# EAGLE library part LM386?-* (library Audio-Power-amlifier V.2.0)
Low Voltage Audio Power Amplifier Source: http://cache.national.com/ds/LM/LM386.pdf
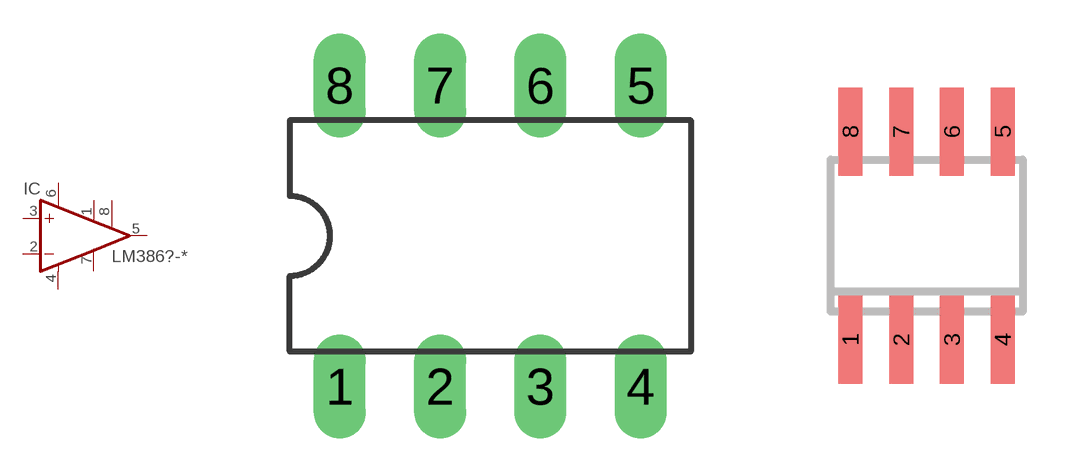
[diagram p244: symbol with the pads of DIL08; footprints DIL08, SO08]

Designator prefix IC

## LM386N-1, LM386N-3, LM386N-4  [DIL08]
1  GAIN  pas
2  -IN  in
3  +IN  in
4  GND  pwr
5  OUT  out
6  VS  pwr
7  BYPASS  pas
8  GAIN  pas

## LM386M-1  [SO08]
Pads as for DIL08

## LM386MM-1  [MMSOP08]
Pads as for DIL08

## LM386NJM386*-  [SIP8]
Pads as for DIL08

## Footprint DIL08 (pad centres in mm)
Dual In Line Package
drill 0.813 pad 1.27 long: 1 -3.81,-3.81; 2 -1.27,-3.81; 3 1.27,-3.81; 4 3.81,-3.81; 5 3.81,3.81; 6 1.27,3.81; 7 -1.27,3.81; 8 -3.81,3.81

## Footprint SO08 (pad centres in mm)
Small Outline Package 8 NS Package M08A
smd 0.6 x 2.2: 1 -1.905,-2.6; 2 -0.635,-2.6; 3 0.635,-2.6; 4 1.905,-2.6; 5 1.905,2.6; 6 0.635,2.6; 7 -0.635,2.6; 8 -1.905,2.6

## Footprint MMSOP08 (pad centres in mm)
Molded Mini Small Outline Package 8 - Lead (0.118" Wide) NS Package Number MUA08A Source: http://cache.national.com/ds/LM/LM386.pdf
smd 0.41 x 1.02: 1 -0.975,-2.4; 2 -0.325,-2.4; 3 0.325,-2.4; 4 0.975,-2.4; 5 0.975,2.4; 6 0.325,2.4; 7 -0.325,2.4; 8 -0.975,2.4

## Footprint SIP8 (pad centres in mm)
drill 0.8 long: 1 -8.8,3.6; 2 -6.3,3.6; 3 -3.8,3.6; 4 -1.4,3.6; 5 1.1,3.6; 6 3.6,3.6; 7 6.1,3.6; 8 8.6,3.6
